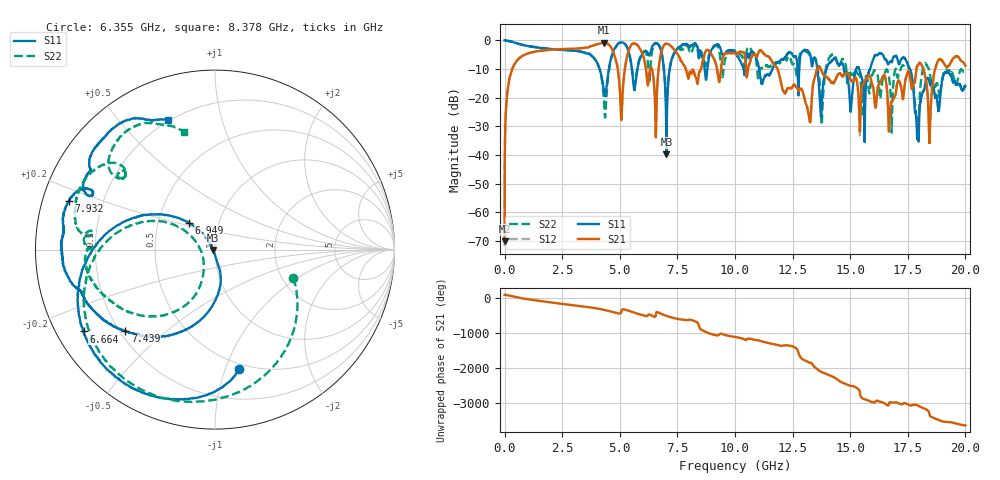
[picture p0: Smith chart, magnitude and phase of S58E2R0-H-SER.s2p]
!{S58E2R0}
!Johanson Technology Inc.
!www.johansontechnology.com
!Test Board Conditions:
!Substrate Type  RO4350B
!Substrate Thickness  60 mil
!Substrate Dk  3.66
!TL Type: GCPW
!TL Trace Width  115 mil
!TL Gap  52 mil
!Electrode orientation  Horizontal
!DUT TOPOLOGY	SERIES
!Mounting Pad LxW  55x428 mil
! Created Tue Apr 13 22:26:00 2021
# hz S ma R 50
! 2 Port Network Data from SP1.SP block
! freq  magS11  angS11  magS21  angS21  magS12  angS12  magS22  angS22
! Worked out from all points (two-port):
!   20001 points, 300 kHz to 20 GHz, reference 50 ohm
!   highest |S21| = -0.79 dB at 4.324 GHz (marker M1); lowest = -70.1 dB at 300 kHz (marker M2)
!   |S21| within 3 dB of the highest: 1.411 GHz to 4.705 GHz (3.294 GHz wide, 108 % of centre); 6.809 GHz to 7.423 GHz (614.1 MHz wide, 8.63 % of centre)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
!   lowest |S11| = -39.7 dB at 7.022 GHz (marker M3), VSWR 1.02, Z = 49 - j0.144 ohm
!   |S11| at or under -10 dB: 11.05 GHz to 11.62 GHz (578 MHz wide, 5.1 % of centre); 14.73 GHz to 15.26 GHz (532.5 MHz wide, 3.55 % of centre); 17.6 GHz to end of sweep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
!   |S22| runs from -32.2 to 0.0 dB; largest |S21 - S12| = 0.014
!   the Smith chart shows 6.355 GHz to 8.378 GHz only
!   S11 on the Smith chart (normalised r, x): 6.355 GHz: 0.46, -1.11; 6.664 GHz: 0.08, -0.28; 6.949 GHz: 0.72, +0.22; 7.439 GHz: 0.22, -0.37; 7.932 GHz: 0.08, +0.16; 8.378 GHz: 0.19, +0.68
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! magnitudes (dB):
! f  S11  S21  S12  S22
! 300 kHz  0.0  -70.1  -71.8  0.0
! 124.3 MHz  -0.1  -17.7  -17.7  -0.1
! 436.3 MHz  -0.7  -8.2  -8.2  -0.7
! 3.334 GHz  -4.0  -2.7  -2.7  -3.9
! 4.324 GHz  -18.3  -0.8  -0.8  -22.7
! 4.962 GHz  -0.9  -13.4  -13.4  -0.9
! 6.355 GHz  -3.4  -9.4  -9.4  -6.7
! 6.664 GHz  -1.3  -11.5  -11.5  -1.4
! 6.667 GHz  -1.3  -11.3  -11.2  -1.4
! 6.949 GHz  -13.6  -1.4  -1.4  -12.6
! 7.022 GHz  -39.7  -1.1  -1.1  -22.3
! 7.439 GHz  -3.4  -4.0  -4.0  -3.7
! 7.932 GHz  -1.3  -12.1  -12.0  -1.9
! 8.378 GHz  -2.3  -15.0  -14.9  -3.3
! 10 GHz  -3.7  -4.4  -4.4  -3.8
! 13.33 GHz  -8.8  -20.2  -20.0  -6.5
! 16.67 GHz  -8.2  -30.2  -30.3  -12.0
! 17.53 GHz  -8.9  -10.7  -10.7  -9.6
! 17.91 GHz  -34.2  -8.9  -8.9  -27.0
! 18.45 GHz  -15.0  -33.2  -32.8  -11.0
! 18.83 GHz  -24.5  -6.8  -6.8  -17.3
! 20 GHz  -15.8  -8.8  -8.8  -10.8
